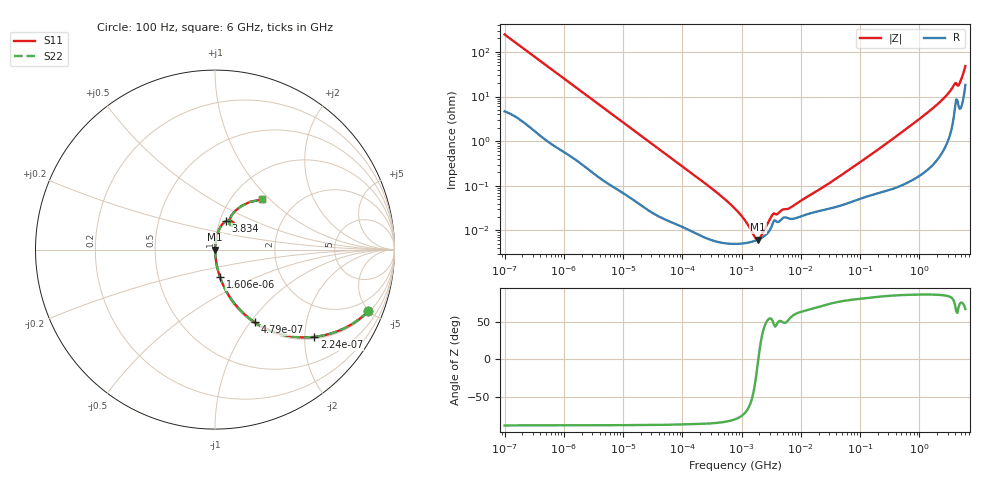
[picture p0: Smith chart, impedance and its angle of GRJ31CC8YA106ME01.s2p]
!Murata Part Number: GRJ31CC8YA106ME01
!These Parameters are Measured in Series Mode Connection
!Data Generated on Jun 19, 2026
!  o--ll--o
!Port1  Port2
!  o------o
!Operation Temp=25[degC], DC Bias Voltage=0[V]
!Freq. Start=100[Hz] Stop=6[GHz] 401[Steps]
# Hz S RI R 50
!Freq.(Hz) S11(Real) S11(Imag) S21(Real) S21(Imag) S12(Real) S12(Imag) S22(Real) S22(Imag)
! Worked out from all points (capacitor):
!   401 points, 100 Hz to 6 GHz, reference 50 ohm
!   read as one part in series: C = 6.43 uF near 109 Hz
!   lowest |Z| = 6.25 mohm at 1.897 MHz (marker M1)
!   series resonance near 1.918 MHz, so ESL is about 1.1 nH
!   S11 on the Smith chart (normalised r, x): 100 Hz: 1.09, -4.92; 224 Hz: 1.05, -2.23; 479 Hz: 1.02, -1.05; 1.606 kHz: 1.01, -0.32; 3.834 GHz: 1.07, +0.35; 6 GHz: 1.37, +0.89
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100  0.8537 -0.3441  0.1463 0.3441  0.1463 0.3441  0.8537 -0.3441
224  0.5533 -0.4862  0.4467 0.4862  0.4467 0.4862  0.5533 -0.4862
479  0.2219 -0.4053  0.7781 0.4053  0.7781 0.4053  0.2219 -0.4053
820  0.0925 -0.2791  0.9075 0.2791  0.9075 0.2791  0.0925 -0.2791
1606  0.0284 -0.1547  0.9716 0.1547  0.9716 0.1547  0.0284 -0.1547
2008  0.0191 -0.1254  0.9809 0.1254  0.9809 0.1254  0.0191 -0.1254
6433  0.00264 -0.0405  0.9974 0.0405  0.9974 0.0405  0.00264 -0.0405
40335  0.000249 -0.00667  0.9998 0.00667  0.9998 0.00667  0.000249 -0.00667
316350  6.1e-05 -0.000861  0.9999 0.000861  0.9999 0.000861  6.1e-05 -0.000861
774597  5e-05 -0.000304  1 0.000304  1 0.000304  5e-05 -0.000304
1449809  5.52e-05 -8.35e-05  0.9999 8.35e-05  0.9999 8.35e-05  5.52e-05 -8.35e-05
1896632  6.24e-05 -3.2e-06  0.9999 3.2e-06  0.9999 3.2e-06  6.24e-05 -3.2e-06
2372521  7.36e-05 6.47e-05  0.9999 -6.47e-05  0.9999 -6.47e-05  7.36e-05 6.47e-05
3394479  0.00015 0.00018  0.9999 -0.00018  0.9999 -0.00018  0.00015 0.00018
6644369  0.000182 0.000267  0.9998 -0.000267  0.9998 -0.000267  0.000182 0.000267
1.555665e7  0.000249 0.000613  0.9998 -0.000613  0.9998 -0.000613  0.000249 0.000613
3.124326e8  0.000902 0.00986  0.9991 -0.00986  0.9991 -0.00986  0.000902 0.00986
1.791126e9  0.00653 0.0577  0.9935 -0.0577  0.9935 -0.0577  0.00653 0.0577
2.802721e9  0.0178 0.0991  0.9822 -0.0991  0.9822 -0.0991  0.0178 0.0991
3.8344e9  0.062 0.159  0.938 -0.159  0.938 -0.159  0.062 0.159
4.796499e9  0.0808 0.1669  0.9192 -0.1669  0.9192 -0.1669  0.0808 0.1669
6e9  0.2604 0.2795  0.7396 -0.2795  0.7396 -0.2795  0.2604 0.2795
